(* Logix 5000 Routine export MTB_Plus_Program; software revision 20.01 *)

TYPE MTB_Config :
STRUCT
   Reserved : INT;
   Pulses_Per_Rev : INT;
   Channel_Mode : INT[30];
   CH32_Analog_1 : INT;
   CH32_Analog_2 : INT;
   Digital_Out_Fault_Mode : SINT;
   Fault_on_Loss_of_Comms : BOOL;
END_STRUCT
END_TYPE

TYPE MTB_Input :
STRUCT
   Digital_Out_Echo : INT;
   Analog_1_Echo : INT;
   Analog_2_Echo : INT;
   Status : INT;
   Channel : REAL[30];
   Speed : REAL;
   Ambient_Temperature : REAL;
   Digital_In : SINT;
END_STRUCT
END_TYPE

TYPE MTB_Channel_Config :
STRUCT
   delta_m : INT;
   delta_b : INT;
END_STRUCT
END_TYPE

TYPE MTB_Output :
STRUCT
   Analog_Out_1 : INT;
   Analog_Out_2 : INT;
   Channel_Config : MTB_Channel_Config[30];
   Status_Control : INT;
   Digital_Out : SINT;
   Fault_Mode : BOOL;
END_STRUCT
END_TYPE

VAR_GLOBAL   (* controller tags *)
   MTB_NFO : MESSAGE;
        MessageParameters(MessageType := Module Reconfigure, RequestedLength := 1, ConnectionPath := MTBPlus)
   MTB_Input : MTB_Input := (Digital_Out_Echo := 145, Analog_2_Echo := 2048, Status := 4363, Channel[0] := 298.0, Channel[1] := 0.12, Channel[2] := 300.0, Channel[3] := 0.01, Channel[4] := 1.0, Channel[5] := 1.0, Channel[7] := -25.0, Channel[25] := -6.2, Channel[26] := -6.2, Channel[27] := 1.0, Channel[28] := 255.0, Channel[29] := 176.0, Ambient_Temperature := 297.4);
   MTB_Config : MTB_Config := (Pulses_Per_Rev := 120, Channel_Mode[0] := 14, Channel_Mode[1] := 8, Channel_Mode[2] := 14, Channel_Mode[3] := 10, Channel_Mode[4] := 15, Channel_Mode[5] := 16, Channel_Mode[7] := 9, Channel_Mode[25] := 1, Channel_Mode[26] := 1, Channel_Mode[28] := 11, Channel_Mode[29] := 12, CH32_Analog_1 := 100, CH32_Analog_2 := 1024, Digital_Out_Fault_Mode := -68, Fault_on_Loss_of_Comms := 1);
   MTB_Output : MTB_Output := (Analog_Out_2 := 2048, Channel_Config[0].delta_m := 2, Channel_Config[0].delta_b := 2, Channel_Config[1].delta_m := 3, Channel_Config[2].delta_b := 2, Channel_Config[28].delta_m := 1, Status_Control := 6, Digital_Out := -111);
   Update_Config : BOOL;
END_VAR

PROGRAM DET_COM

ROUTINE MTB_Plus_Program   (* ladder *)
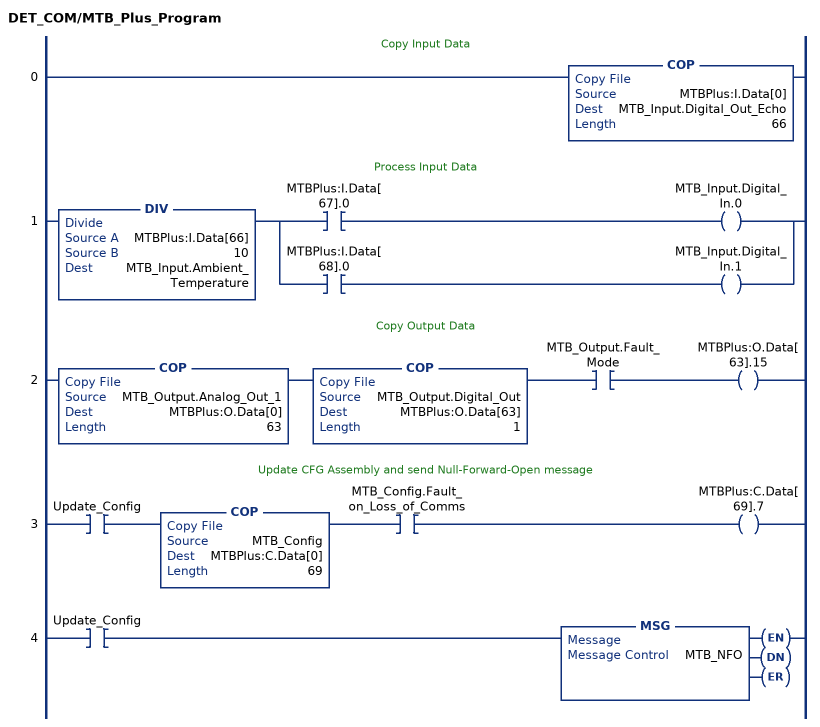
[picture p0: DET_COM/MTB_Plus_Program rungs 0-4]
   // Copy Input Data
   0: COP(MTBPlus:I.Data[0],MTB_Input.Digital_Out_Echo,66);
   // Process Input Data
   1: DIV(MTBPlus:I.Data[66],10,MTB_Input.Ambient_Temperature)[XIC(MTBPlus:I.Data[67].0) OTE(MTB_Input.Digital_In.0) ,XIC(MTBPlus:I.Data[68].0) OTE(MTB_Input.Digital_In.1) ];
   // Copy Output Data
   2: COP(MTB_Output.Analog_Out_1,MTBPlus:O.Data[0],63)COP(MTB_Output.Digital_Out,MTBPlus:O.Data[63],1)XIC(MTB_Output.Fault_Mode)OTE(MTBPlus:O.Data[63].15);
   // Update CFG Assembly and send Null-Forward-Open message
   3: XIC(Update_Config)COP(MTB_Config,MTBPlus:C.Data[0],69)XIC(MTB_Config.Fault_on_Loss_of_Comms)OTE(MTBPlus:C.Data[69].7);
   4: XIC(Update_Config)MSG(MTB_NFO);
END_ROUTINE
END_PROGRAM
